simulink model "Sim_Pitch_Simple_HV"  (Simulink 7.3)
settings: Solver=ode23s  StartTime=0.0  StopTime=300  RelTol=1e-3
InitFcn:
  | init
StartFcn:
  | init
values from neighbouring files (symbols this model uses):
  d2r = pi/180    (= 0.0174532925199)    [init.m]    (also in robust.m)
  r2d = 180/pi    (= 57.2957795131)    [init.m]    (also in robust.m)
undefined symbols (not defined in the file or in its folder): Apa, Bpa, Cpa, Dpa, Kmix, Kq

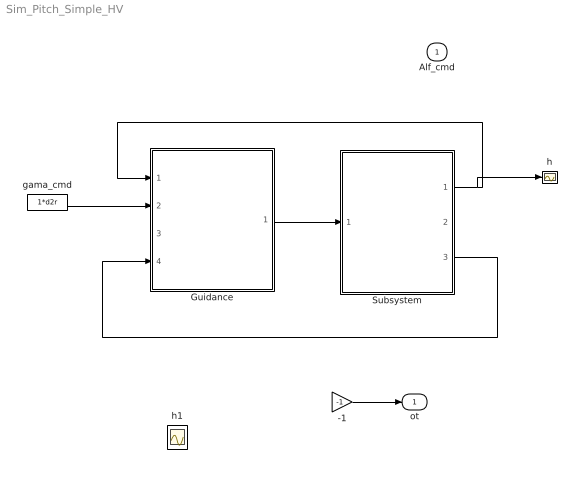
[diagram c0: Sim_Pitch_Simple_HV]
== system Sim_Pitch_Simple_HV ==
  Alf_cmd : Inport  OutDataType=sfix(16)  OutScaling=2^0
  -1 : Gain  Gain=-1  ParameterDataType=sfix(16)  ParameterScaling=2^0  OutDataType=sfix(16)  OutScaling=2^0
  Guidance : Subsystem
  Subsystem : Subsystem
  gama_cmd : Constant  Value=1*d2r  OutDataType=sfix(16)  OutScaling=2^0
  h : Scope
  h1 : Scope
  ot : Outport  OutDataType=sfix(16)  OutScaling=2^0
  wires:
  Subsystem/1(h) -> Guidance/1(h), h/1
  gama_cmd/1 -> Guidance/2(gamma_cmd)
  Subsystem/3(hdot) -> Guidance/4(hdot)
  -1/1 -> ot/1
  Guidance/1(Nz_cmd) -> Subsystem/1(Alf_cmd)

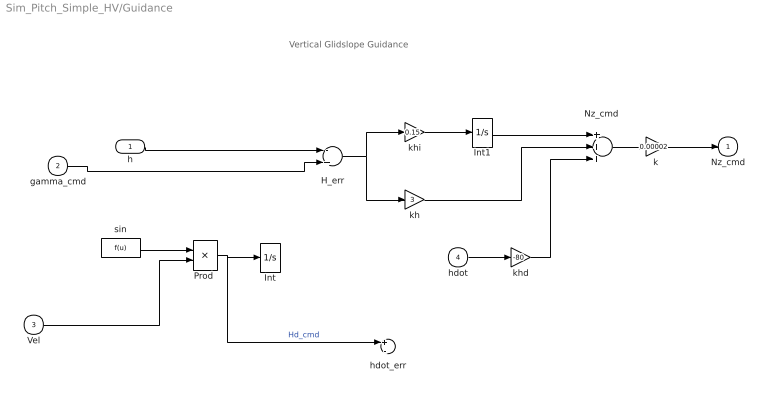
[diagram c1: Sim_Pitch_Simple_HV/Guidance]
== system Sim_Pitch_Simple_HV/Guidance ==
  note: Vertical Glidslope Guidance
  h : Inport  OutDataType=sfix(16)  OutScaling=2^0
  gamma_cmd : Inport  Port=2  OutDataType=sfix(16)  OutScaling=2^0
  Vel : Inport  Port=3  OutDataType=sfix(16)  OutScaling=2^0
  hdot : Inport  Port=4  OutDataType=sfix(16)  OutScaling=2^0
  H_err : Sum  Inputs=-+  OutDataType=sfix(16)  OutScaling=2^0
  Int : Integrator
  Int1 : Integrator
  "Nz_cmd " : Sum  Inputs=+++  OutDataType=sfix(16)  OutScaling=2^0
  "Prod " : Product  OutDataType=sfix(16)  OutScaling=2^0
  hdot_err : Sum  Inputs=+-  OutDataType=sfix(16)  OutScaling=2^0
  k : Gain  Gain=0.00002  ParameterDataType=sfix(16)  ParameterScaling=2^0  OutDataType=sfix(16)  OutScaling=2^0
  kh : Gain  Gain=3  ParameterDataType=sfix(16)  ParameterScaling=2^0  OutDataType=sfix(16)  OutScaling=2^0
  khd : Gain  Gain=-80  ParameterDataType=sfix(16)  ParameterScaling=2^0  OutDataType=sfix(16)  OutScaling=2^0
  khi : Gain  Gain=0.15  ParameterDataType=sfix(16)  ParameterScaling=2^0  OutDataType=sfix(16)  OutScaling=2^0
  sin : Fcn
  Nz_cmd : Outport  InitialOutput=0
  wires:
  "Nz_cmd "/1 -> k/1
  h/1 -> H_err/1
  sin/1 -> "Prod "/1
  "Prod "/1 -> Int/1, hdot_err/1  "Hd_cmd"
  Vel/1 -> "Prod "/2
  khi/1 -> Int1/1
  H_err/1 -> khi/1, kh/1
  Int1/1 -> "Nz_cmd "/1
  kh/1 -> "Nz_cmd "/2
  k/1 -> Nz_cmd/1
  gamma_cmd/1 -> H_err/2
  hdot/1 -> khd/1
  khd/1 -> "Nz_cmd "/3

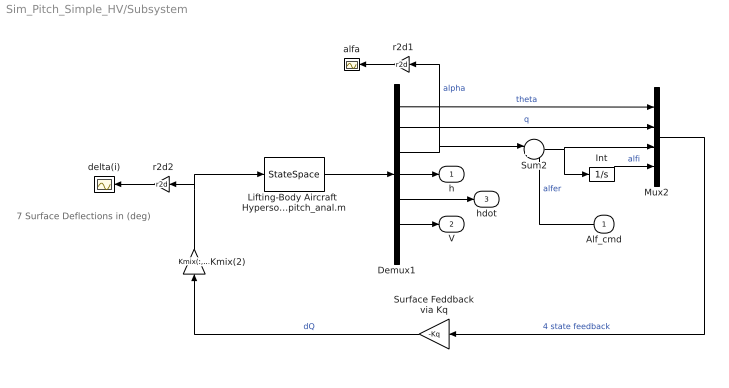
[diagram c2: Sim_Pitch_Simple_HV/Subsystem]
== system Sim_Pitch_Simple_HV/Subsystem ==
  note: 7 Surface Deflections in (deg)
  Alf_cmd : Inport  OutDataType=sfix(16)  OutScaling=2^0
  " r2d1" : Gain  Gain=r2d  ParameterDataType=sfix(16)  ParameterScaling=2^0  OutDataType=sfix(16)  OutScaling=2^0
  " r2d2" : Gain  Gain=r2d  ParameterDataType=sfix(16)  ParameterScaling=2^0  OutDataType=sfix(16)  OutScaling=2^0
  Demux1 : Demux  Outputs=7
  Int : Integrator
  Kmix(2) : Gain  Gain=Kmix(:,2)  Multiplication=Matrix(K*u)  ParameterDataType=sfix(16)  ParameterScaling=2^0  OutDataType=sfix(16)  OutScaling=2^0
  Lifting-Body Aircraft  Hypersonic Pitch  Analysis Model from file pitch_anal.m : StateSpace  A=Apa  B=Bpa  C=Cpa  D=Dpa
  Mux2 : Mux
  Sum2 : Sum  Inputs=|+-  OutDataType=sfix(16)  OutScaling=2^0
  Surface Feddback via Kq : Gain  Gain=-Kq  Multiplication=Matrix(K*u)  ParameterDataType=sfix(16)  ParameterScaling=2^0  OutDataType=sfix(16)  OutScaling=2^0
  alfa : Scope
  delta(i) : Scope
  h : Outport  OutDataType=sfix(16)  OutScaling=2^0
  V : Outport  Port=2  OutDataType=sfix(16)  OutScaling=2^0
  hdot : Outport  Port=3  OutDataType=sfix(16)  OutScaling=2^0
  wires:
  Mux2/1 -> Surface Feddback via Kq/1  "4 state feedback"
  Surface Feddback via Kq/1 -> Kmix(2)/1  "dQ"
  Lifting-Body Aircraft  Hypersonic Pitch  Analysis Model from file pitch_anal.m/1 -> Demux1/1
  " r2d1"/1 -> alfa/1
  Kmix(2)/1 -> Lifting-Body Aircraft  Hypersonic Pitch  Analysis Model from file pitch_anal.m/1, " r2d2"/1
  " r2d2"/1 -> delta(i)/1
  Demux1/1 -> Mux2/1  "theta"
  Demux1/2 -> Mux2/2  "q"
  Int/1 -> Mux2/4  "alfi"
  Demux1/3 -> " r2d1"/1, Sum2/1  "alpha"
  Demux1/6 -> V/1
  Demux1/5 -> hdot/1
  Demux1/4 -> h/1
  Sum2/1 -> Mux2/3, Int/1
  Alf_cmd/1 -> Sum2/2  "alfer"
